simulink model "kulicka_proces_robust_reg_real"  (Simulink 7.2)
libraries: mathlib x44, anallib x4, reglib x3, inoutlib x2, arclib x1

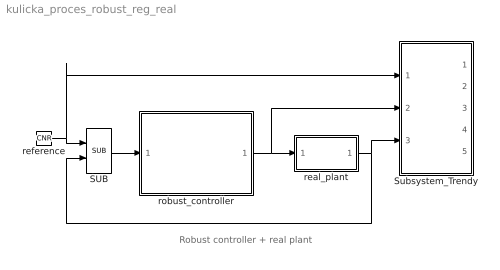
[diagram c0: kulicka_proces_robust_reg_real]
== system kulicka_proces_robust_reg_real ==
  note: Robust controller + real plant
  SUB : mathlib/SUB  SystemSampleTime=-1
  Subsystem_Trendy : Subsystem
  real_plant : Subsystem
  reference : mathlib/CNR  ycn=0.3
  robust_controller : Subsystem
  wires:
  SUB/1 -> robust_controller/1(e)
  real_plant/1(y) -> SUB/2, Subsystem_Trendy/3(y_out)
  reference/1 -> SUB/1, Subsystem_Trendy/1(w_in)
  robust_controller/1(u) -> Subsystem_Trendy/2(u_out), real_plant/1(u)

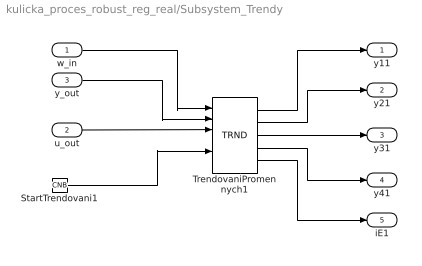
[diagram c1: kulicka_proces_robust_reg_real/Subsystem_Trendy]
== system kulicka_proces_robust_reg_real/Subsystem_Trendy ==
  w_in : Inport  Port=1
  u_out : Inport  Port=2
  y_out : Inport  Port=3
  StartTrendovani1 : mathlib/CNB  SystemSampleTime=-1  YCN=on
  TrendovaniPromennych1 : arclib/TRND  SystemSampleTime=-1  n=4  l=2000  btype=8: Double  ptype1=1: Store  ptype2=1: Store  ptype3=1: Store  ptype4=1: Store  pfac=1  afac=0  arc=2  id=1  Title=Trend Title
  y11 : Outport  Port=1
  y21 : Outport  Port=2
  y31 : Outport  Port=3
  y41 : Outport  Port=4
  iE1 : Outport  Port=5
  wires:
  StartTrendovani1/1 -> TrendovaniPromennych1/5
  TrendovaniPromennych1/1 -> y11/1
  TrendovaniPromennych1/2 -> y21/1
  TrendovaniPromennych1/3 -> y31/1
  TrendovaniPromennych1/4 -> y41/1
  TrendovaniPromennych1/5 -> iE1/1
  u_out/1 -> TrendovaniPromennych1/3
  w_in/1 -> TrendovaniPromennych1/1
  y_out/1 -> TrendovaniPromennych1/2

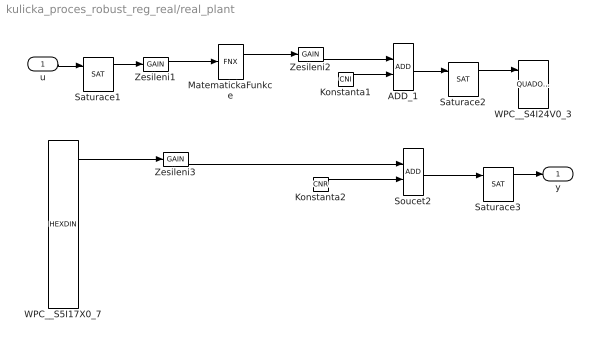
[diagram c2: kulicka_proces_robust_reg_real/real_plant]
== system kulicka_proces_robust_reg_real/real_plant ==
  u : Inport  Port=1
  ADD_1 : mathlib/ADD  SystemSampleTime=-1
  Konstanta1 : mathlib/CNI  SystemSampleTime=-1  ycn=5
  Konstanta2 : mathlib/CNR  SystemSampleTime=-1  ycn=0.96
  MatematickaFunkce : mathlib/FNX  SystemSampleTime=-1  ifn=2: asin  yerr=0
  Saturace1 : reglib/SAT  SystemSampleTime=-1  tp=1  tn=1  hilim0=0.01  lolim0=-0.01  HLD=on
  Saturace2 : reglib/SAT  SystemSampleTime=-1  tp=1  tn=1  hilim0=10  lolim0=0  HLD=on
  Saturace3 : reglib/SAT  SystemSampleTime=-1  tp=1  tn=1  hilim0=0.95  lolim0=0  HLD=on
  Soucet2 : mathlib/ADD  SystemSampleTime=-1
  WPC__S4I24V0_3 : inoutlib/QUADOUT  SystemSampleTime=-1
  WPC__S5I17X0_7 : inoutlib/HEXDIN  SystemSampleTime=-1
  Zesileni1 : mathlib/GAIN  SystemSampleTime=-1  k=50
  Zesileni2 : mathlib/GAIN  SystemSampleTime=-1  k=9.5493
  Zesileni3 : mathlib/GAIN  SystemSampleTime=-1  k=-0.1
  y : Outport  Port=1
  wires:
  ADD_1/1 -> Saturace2/1
  Konstanta1/1 -> ADD_1/2
  Konstanta2/1 -> Soucet2/2
  MatematickaFunkce/1 -> Zesileni2/1
  Saturace1/1 -> Zesileni1/1
  Saturace2/1 -> WPC__S4I24V0_3/1
  Saturace3/1 -> y/1
  Soucet2/1 -> Saturace3/1
  WPC__S5I17X0_7/2 -> Zesileni3/1
  Zesileni1/1 -> MatematickaFunkce/1
  Zesileni2/1 -> ADD_1/1
  Zesileni3/1 -> Soucet2/1
  u/1 -> Saturace1/1

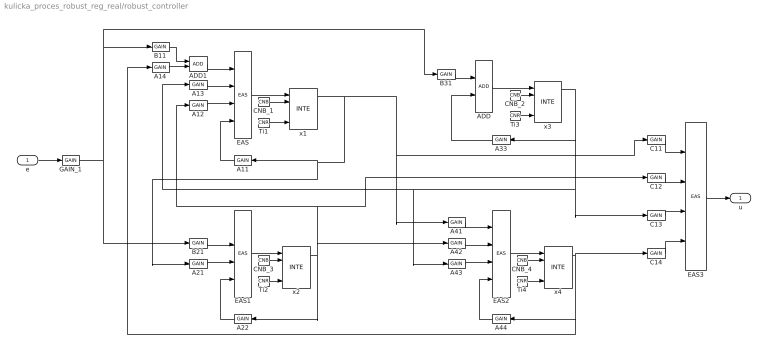
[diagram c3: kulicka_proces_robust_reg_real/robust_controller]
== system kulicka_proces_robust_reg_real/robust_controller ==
  e : Inport  Port=1
  A11 : mathlib/GAIN  Orientation=left  SystemSampleTime=-1  k=-0.3206
  A12 : mathlib/GAIN  SystemSampleTime=-1  k=-818.6
  A13 : mathlib/GAIN  SystemSampleTime=-1  k=-0.1872
  A14 : mathlib/GAIN  SystemSampleTime=-1  k=14.99
  A21 : mathlib/GAIN  SystemSampleTime=-1  k=0.0009766
  A22 : mathlib/GAIN  Orientation=left  SystemSampleTime=-1  k=-1.194
  A33 : mathlib/GAIN  Orientation=left  SystemSampleTime=-1  k=-0.00025
  A41 : mathlib/GAIN  SystemSampleTime=-1  k=-20.45
  A42 : mathlib/GAIN  SystemSampleTime=-1  k=-5679
  A43 : mathlib/GAIN  SystemSampleTime=-1  k=-11.98
  A44 : mathlib/GAIN  Orientation=left  SystemSampleTime=-1  k=-40.8
  ADD : mathlib/ADD  SystemSampleTime=-1
  ADD1 : mathlib/ADD  SystemSampleTime=-1
  B11 : mathlib/GAIN  SystemSampleTime=-1  k=-1067
  B21 : mathlib/GAIN  SystemSampleTime=-1  k=-1.745
  B31 : mathlib/GAIN  SystemSampleTime=-1  k=-83.5
  C11 : mathlib/GAIN  SystemSampleTime=-1  k=-0.0000299
  C12 : mathlib/GAIN  SystemSampleTime=-1  k=-0.008302
  C13 : mathlib/GAIN  SystemSampleTime=-1  k=-0.00001751
  C14 : mathlib/GAIN  SystemSampleTime=-1  k=0.001402
  CNB_{1..4} (4 alike) : mathlib/CNB  YCN=on
  EAS{,1..3} (4 alike) : mathlib/EAS  SystemSampleTime=-1  a=1  b=1  c=1  d=1  y0=0
  GAIN_1 : mathlib/GAIN  SystemSampleTime=-1  k=1
  Ti{1..4} (4 alike) : mathlib/CNR  ycn=1
  x{1..4} (4 alike) : anallib/INTE  ymin=-1  ymax=1
  u : Outport  Port=1
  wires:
  A11/1 -> EAS/4
  A12/1 -> EAS/3
  A13/1 -> EAS/2
  A14/1 -> ADD1/2
  A21/1 -> EAS1/3
  A22/1 -> EAS1/4
  A33/1 -> ADD/2
  A41/1 -> EAS2/1
  A42/1 -> EAS2/2
  A43/1 -> EAS2/3
  A44/1 -> EAS2/4
  ADD/1 -> x3/1
  ADD1/1 -> EAS/1
  B11/1 -> ADD1/1
  B21/1 -> EAS1/2
  B31/1 -> ADD/1
  C11/1 -> EAS3/1
  C12/1 -> EAS3/2
  C13/1 -> EAS3/3
  C14/1 -> EAS3/4
  CNB_1/1 -> x1/2
  CNB_2/1 -> x3/2
  CNB_3/1 -> x2/2
  CNB_4/1 -> x4/2
  EAS/1 -> x1/1
  EAS1/1 -> x2/1
  EAS2/1 -> x4/1
  EAS3/1 -> u/1
  GAIN_1/1 -> B21/1, B11/1, B31/1
  Ti1/1 -> x1/5
  Ti2/1 -> x2/5
  Ti3/1 -> x3/5
  Ti4/1 -> x4/5
  e/1 -> GAIN_1/1
  x1/1 -> A41/1, C11/1, A11/1, A21/1
  x2/1 -> A22/1, A42/1, A12/1, C12/1
  x3/1 -> A33/1, C13/1, A13/1, A43/1
  x4/1 -> C14/1, A14/1, A44/1
